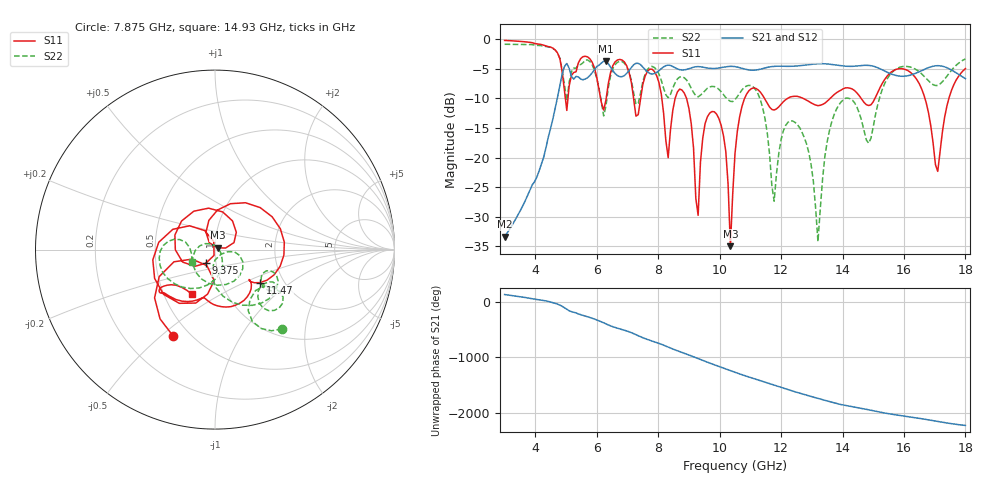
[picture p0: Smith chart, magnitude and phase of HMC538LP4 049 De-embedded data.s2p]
! Chelmsford, MA 01824
! http://www.hittite.com
! Tel: 978-250-3343
! Fax: 978-250-3373
! Device  :  HMC538LP4
! Description:  600 Analog Phase Shifter
! Frequency  :  6.0 GHz - 15.0 GHz
! Package  :  LP4  - 4x4 mm Quad Flatpack No-Lead (QFN) Plastic Package: 24 pin
! Ports  :  2 RF, 1 DC
!  Pin  3  = Rfin  = Port 1
!  Pin  16  = Rfout = Port 2
!  pin  21  = vCTL
! Voltages:  VCTL  = 0 to 5.0 Volts
! Currents :  Vb(V)  Vd(V)  Ib(mA)  Id(mA)
!  0.00  4.90  0.000000	0.477956
! Data:  The device was measured on evaluation board 111296-1.
!  Data was collected using a calibrated network analyzer.
!  The evaluation circuit board was modeled and simulated.This was use
!  to removed the evaluation board circuit from the measured data.
!  The reference plane is the center of the package pin.
! Misc:  Lot #
!Date Measured:  03 - 11 -2009
! Date:  03 - 17 -2009
! Note:
!  Hittite Microwave supplies this data as a sample of measured data at the
!  package pin for this package product.  Your particular data for this product
!  may vary.
!  Data was taken at 25 degrees C.
!  Hittite Microwave reserves the right to change this data at anytime.
# MHz S MA R 50
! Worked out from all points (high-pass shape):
!   201 points, 3 GHz to 18 GHz, reference 50 ohm
!   highest |S21| = -3.67 dB at 6.3 GHz (marker M1); lowest = -33.4 dB at 3 GHz (marker M2)
!   |S21| within 3 dB of the highest: 4.842 GHz to 5.242 GHz (400.2 MHz wide, 7.94 % of centre); 5.636 GHz to end of sweep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
!   lowest |S11| = -35.0 dB at 10.35 GHz (marker M3), VSWR 1.04, Z = 51.5 + j1.04 ohm
!   |S11| at or under -10 dB: 8.924 GHz to 10.81 GHz (1.887 GHz wide, 19.1 % of centre); 11.46 GHz to 12.21 GHz (747.8 MHz wide, 6.32 % of centre); 12.73 GHz to 13.59 GHz (867.6 MHz wide, 6.59 % of centre)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
!   |S22| runs from -34.2 to -0.8 dB; largest |S21 - S12| = 0.0023
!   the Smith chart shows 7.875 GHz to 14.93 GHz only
!   S11 on the Smith chart (normalised r, x): 7.875 GHz: 0.41, -0.55; 9.375 GHz: 0.89, -0.14; 11.47 GHz: 1.52, -0.62; 14.93 GHz: 0.69, -0.37
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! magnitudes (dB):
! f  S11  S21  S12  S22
! 3 GHz  -0.2  -33.4  -33.4  -0.8
! 5.55 GHz  -2.9  -6.8  -6.8  -4.0
! 6.3 GHz  -10.2  -3.7  -3.7  -11.2
! 7.875 GHz  -5.4  -5.8  -5.8  -4.8
! 8.025 GHz  -7.3  -5.3  -5.3  -5.9
! 8.325 GHz  -20.0  -4.3  -4.4  -9.9
! 8.925 GHz  -10.0  -5.1  -5.1  -6.9
! 9.3 GHz  -29.8  -4.6  -4.6  -9.7
! 9.375 GHz  -20.8  -4.6  -4.6  -9.4
! 9.975 GHz  -13.4  -4.8  -4.9  -8.5
! 10.35 GHz  -35.0  -4.6  -4.6  -10.5
! 10.5 GHz  -19.3  -4.6  -4.6  -10.2
! 11.47 GHz  -10.1  -4.8  -4.8  -13.3
! 11.78 GHz  -11.9  -4.6  -4.6  -27.4
! 12.3 GHz  -9.7  -4.6  -4.6  -13.8
! 13.05 GHz  -10.9  -4.2  -4.2  -24.0
! 13.2 GHz  -11.2  -4.1  -4.1  -34.2
! 13.8 GHz  -9.0  -4.3  -4.4  -11.8
! 14.93 GHz  -11.1  -4.4  -4.5  -16.7
! 15.53 GHz  -5.8  -5.7  -5.7  -6.1
! 17.1 GHz  -22.3  -4.4  -4.5  -7.8
! 18 GHz  -4.9  -6.6  -6.6  -3.3
